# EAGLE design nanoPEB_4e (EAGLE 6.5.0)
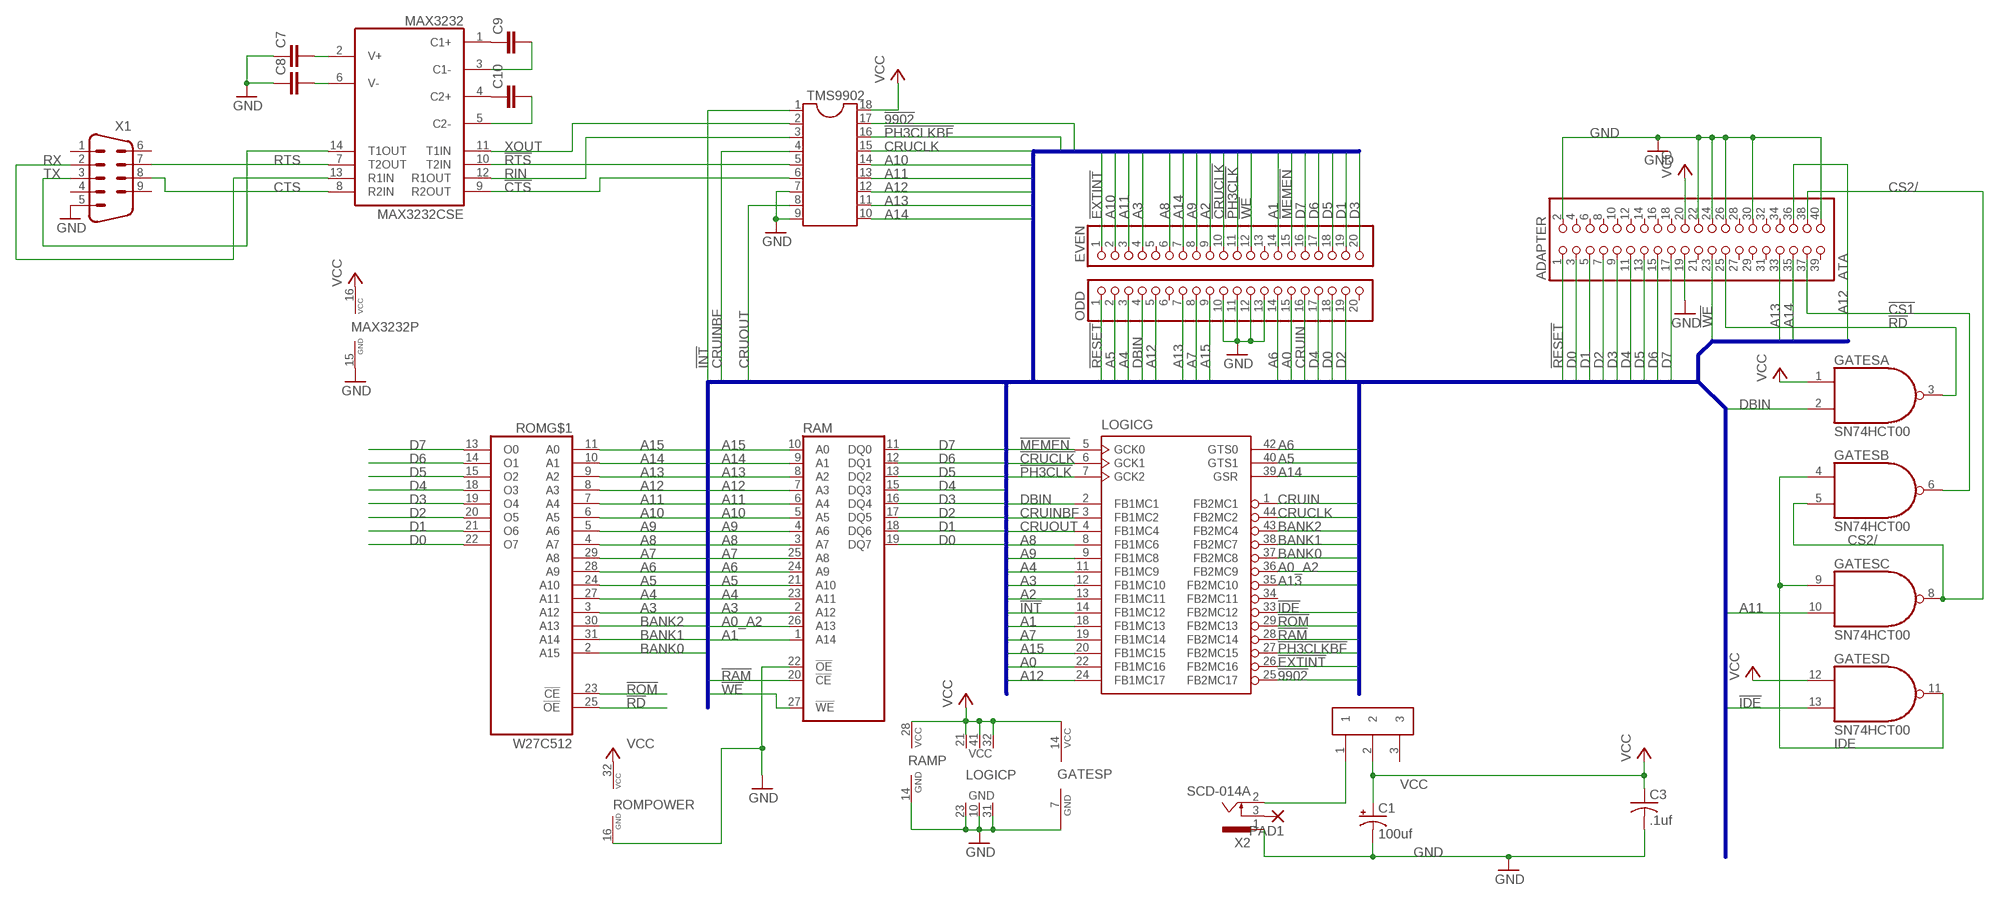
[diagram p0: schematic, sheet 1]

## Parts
ADAPTER  ATA  PINHD-2X20  [2X20]
C1  100uf  CPOL-USE2.5-6  [E2,5-6]
C3  .1uf  C-USC0805  [C0805]
C7  C-EUC0805  [C0805]
C8  C-EUC0805  [C0805]
C9  C-EUC0805  [C0805]
C10  C-EUC0805  [C0805]
EVEN  PINHD-1X20  [1X20]
GATES  SN74HCT00  74LS00D  [SO14]
LOGIC  XC9536-44PC44  [PC44]
MAX3232  MAX3232CSE  [SO16]
ODD  PINHD-1X20  [1X20]
PAD1  1,6/0,8  [1,6/0,8]
POWER  OS1020  [OS1020]
RAM  LH52256CHN  [SOP28]
ROM  W27C512  [PLCC32R-WINBOND]
TMS9902  DIL18S  [SOCKED-18]
X1  M09H  [M09H]
X2  SCD-014A  [SCD-014-A]

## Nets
!9902: LOGIC.25(G:FB2MC17) TMS9902.17
!CRUCLK: EVEN.10 LOGIC.6(G:GCK1)
!CS1: ADAPTER.37 GATES.6(B:O)
!CTS: MAX3232.9(R2OUT) TMS9902.6
!EXTINT: EVEN.1 LOGIC.26(G:FB2MC16)
!IDE: GATES.13(D:I1) LOGIC.33(G:FB2MC12)
!INT: LOGIC.14(G:FB1MC12) TMS9902.1
!MEMEN: EVEN.15 LOGIC.5(G:GCK0)
!PH3CLK: EVEN.11 LOGIC.7(G:GCK2)
!PH3CLKBF: LOGIC.27(G:FB2MC15) TMS9902.16
!RAM: LOGIC.28(G:FB2MC14) RAM.20(!CE)
!RD: ADAPTER.25 GATES.3(A:O) ROM.25(!OE)
!RESET: ADAPTER.1 ODD.1
!ROM: LOGIC.29(G:FB2MC13) ROM.23(!CE)
!RTS: MAX3232.10(T2IN) TMS9902.5
!WE: ADAPTER.23 EVEN.12 RAM.27(!WE)
A0: LOGIC.22(G:FB1MC16) ODD.15
A0_A2: LOGIC.36(G:FB2MC9) RAM.26(A13)
A1: EVEN.14 LOGIC.18(G:FB1MC13) RAM.1(A14)
A2: EVEN.9 LOGIC.13(G:FB1MC11)
A3: EVEN.4 LOGIC.12(G:FB1MC10) RAM.2(A12) ROM.3(A12)
A4: LOGIC.11(G:FB1MC9) ODD.3 RAM.23(A11) ROM.27(A11)
A5: LOGIC.40(G:GTS1) ODD.2 RAM.21(A10) ROM.24(A10)
A6: LOGIC.42(G:GTS0) ODD.14 RAM.24(A9) ROM.28(A9)
A7: LOGIC.19(G:FB1MC14) ODD.8 RAM.25(A8) ROM.29(A8)
A8: EVEN.6 LOGIC.8(G:FB1MC6) RAM.3(A7) ROM.4(A7)
A9: EVEN.8 LOGIC.9(G:FB1MC8) RAM.4(A6) ROM.5(A6)
A10: EVEN.2 RAM.5(A5) ROM.6(A5) TMS9902.14
A11: EVEN.3 GATES.10(C:I1) RAM.6(A4) ROM.7(A4) TMS9902.13
A12: ADAPTER.36 LOGIC.24(G:FB1MC17) ODD.5 RAM.7(A3) ROM.8(A3) TMS9902.12
A13: ADAPTER.33 LOGIC.35(G:FB2MC10) ODD.7 RAM.8(A2) ROM.9(A2) TMS9902.11
A14: ADAPTER.35 EVEN.7 LOGIC.39(G:GSR) RAM.9(A1) ROM.10(A1) TMS9902.10
A15: LOGIC.20(G:FB1MC15) ODD.9 RAM.10(A0) ROM.11(A0)
BANK0: LOGIC.37(G:FB2MC8) ROM.2(A15)
BANK1: LOGIC.38(G:FB2MC7) ROM.31(A14)
BANK2: LOGIC.43(G:FB2MC4) ROM.30(A13)
CRUCLK: LOGIC.44(G:FB2MC2) TMS9902.15
CRUIN: LOGIC.1(G:FB2MC1) ODD.16
CRUINBF: LOGIC.3(G:FB1MC2) TMS9902.4
CRUOUT: LOGIC.4(G:FB1MC4) TMS9902.8
CS2/: ADAPTER.38 GATES.5(B:I1) GATES.8(C:O)
CTS: MAX3232.8(R2IN) X1.8
D0: ADAPTER.3 ODD.18 RAM.19(DQ7) ROM.22(O7)
D1: ADAPTER.5 EVEN.19 RAM.18(DQ6) ROM.21(O6)
D2: ADAPTER.7 ODD.19 RAM.17(DQ5) ROM.20(O5)
D3: ADAPTER.9 EVEN.20 RAM.16(DQ4) ROM.19(O4)
D4: ADAPTER.11 ODD.17 RAM.15(DQ3) ROM.18(O3)
D5: ADAPTER.13 EVEN.18 RAM.13(DQ2) ROM.15(O2)
D6: ADAPTER.15 EVEN.17 RAM.12(DQ1) ROM.14(O1)
D7: ADAPTER.17 EVEN.16 RAM.11(DQ0) ROM.13(O0)
DBIN: GATES.2(A:I1) LOGIC.2(G:FB1MC1) ODD.4
GND [gnd]: ADAPTER.2 ADAPTER.19 ADAPTER.22 ADAPTER.24 ADAPTER.26 ADAPTER.30 ADAPTER.40 C1.- C3.2 C7.1 C8.1 GATES.7(P:GND) LOGIC.10(P:GND) LOGIC.23(P:GND) LOGIC.31(P:GND) MAX3232.15(GND) ODD.10 ODD.11 ODD.12 ODD.13 RAM.14(GND) RAM.22(!OE) ROM.16(POWER:GND) TMS9902.7 TMS9902.9 X1.5 X2.1
IDE: GATES.4(B:I0) GATES.9(C:I0) GATES.11(D:O)
N$1: C9.1 MAX3232.1(C1+)
N$2: C9.2 MAX3232.3(C1-)
N$3: C10.1 MAX3232.4(C2+)
N$5: PAD1.1(P) X2.3
N$6: POWER.1 X2.2
N$7: C8.2 MAX3232.6(V-)
N$8: C7.2 MAX3232.2(V+)
N$9: C10.2 MAX3232.5(C2-)
RIN: MAX3232.12(R1OUT) TMS9902.3
RTS: MAX3232.7(T2OUT) X1.7
RX: MAX3232.13(R1IN) X1.2
TX: MAX3232.14(T1OUT) X1.3
VCC [VCC]: ADAPTER.20 C1.+ C3.1 GATES.1(A:I0) GATES.12(D:I0) GATES.14(P:VCC) LOGIC.21(P:VCC) LOGIC.32(P:VCC) LOGIC.41(P:VCC) MAX3232.16(VCC) POWER.2 RAM.28(VCC) ROM.32(POWER:VCC) TMS9902.18
XOUT: MAX3232.11(T1IN) TMS9902.2
Unconnected: ADAPTER.4 ADAPTER.6 ADAPTER.8 ADAPTER.10 ADAPTER.12 ADAPTER.14 ADAPTER.16 ADAPTER.18 ADAPTER.21 ADAPTER.27 ADAPTER.28 ADAPTER.29 ADAPTER.31 ADAPTER.32 ADAPTER.34 ADAPTER.39 EVEN.5 EVEN.13 LOGIC.15(J:TDI) LOGIC.16(J:TMS) LOGIC.17(J:TCK) LOGIC.30(J:TDO) LOGIC.34(G:FB2MC11) ODD.6 ODD.20 POWER.3 ROM.1(NC1:NC) ROM.12(NC2:NC) ROM.17(NC3:NC) ROM.26(NC4:NC) X1.1 X1.4 X1.6 X1.9

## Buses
A[0..15],D[0..7],!MEMEN,!CRUCLK,CRUIN,!WE,DBIN,!IDE,!RAM,!ROM,!WE,A0_A2,BANK[0..2],!RESET,!9902,!EXTINT,!PH3CLK,!PH3CLKBF,CRUOUT,CRUCLK,CRUINBF,!INT

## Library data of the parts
ADAPTER = pinhead:PINHD-2X20: PIN HEADER
C1 = rcl:CPOL-US: POLARIZED CAPACITOR, American symbol
C3 = rcl:C-US: CAPACITOR, American symbol
C7-C10 = rcl:C-EU: CAPACITOR, European symbol
EVEN ODD = pinhead:PINHD-1X20: PIN HEADER
GATES = 74xx-us:74*00: Quad 2-input NAND gate
LOGIC = xilinx:XC9536-44
MAX3232 = maxim:MAX3232*: True RS-232 Transceivers 3.0V to 5.5V, Low-Power up to 1Mbps, Using Four 0.1µF External Capacitors Source: http://pdfserv.maxim-ic.com/en/ds/MAX3222-MAX3241.pdf; MPN: MAX3232CSE; OC_FARNELL: 9725490; OC_NEWARK: 90C2890
PAD1 = wirepad:1,6/0,8: THROUGH-HOLE PAD
POWER = OS1020:OS1020
RAM = memory-sram:LH52256CHN: MEMORY
ROM = am29-memory:W27C512
TMS9902 = ic-package:DIL18: Dual In Line
X1 = con-subd:M09: SUB-D
X2 = power_jack:SCD-014A: Power Jack 2.1mm

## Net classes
1 gnd: width 0.406 mm
2 VCC: width 0.406 mm

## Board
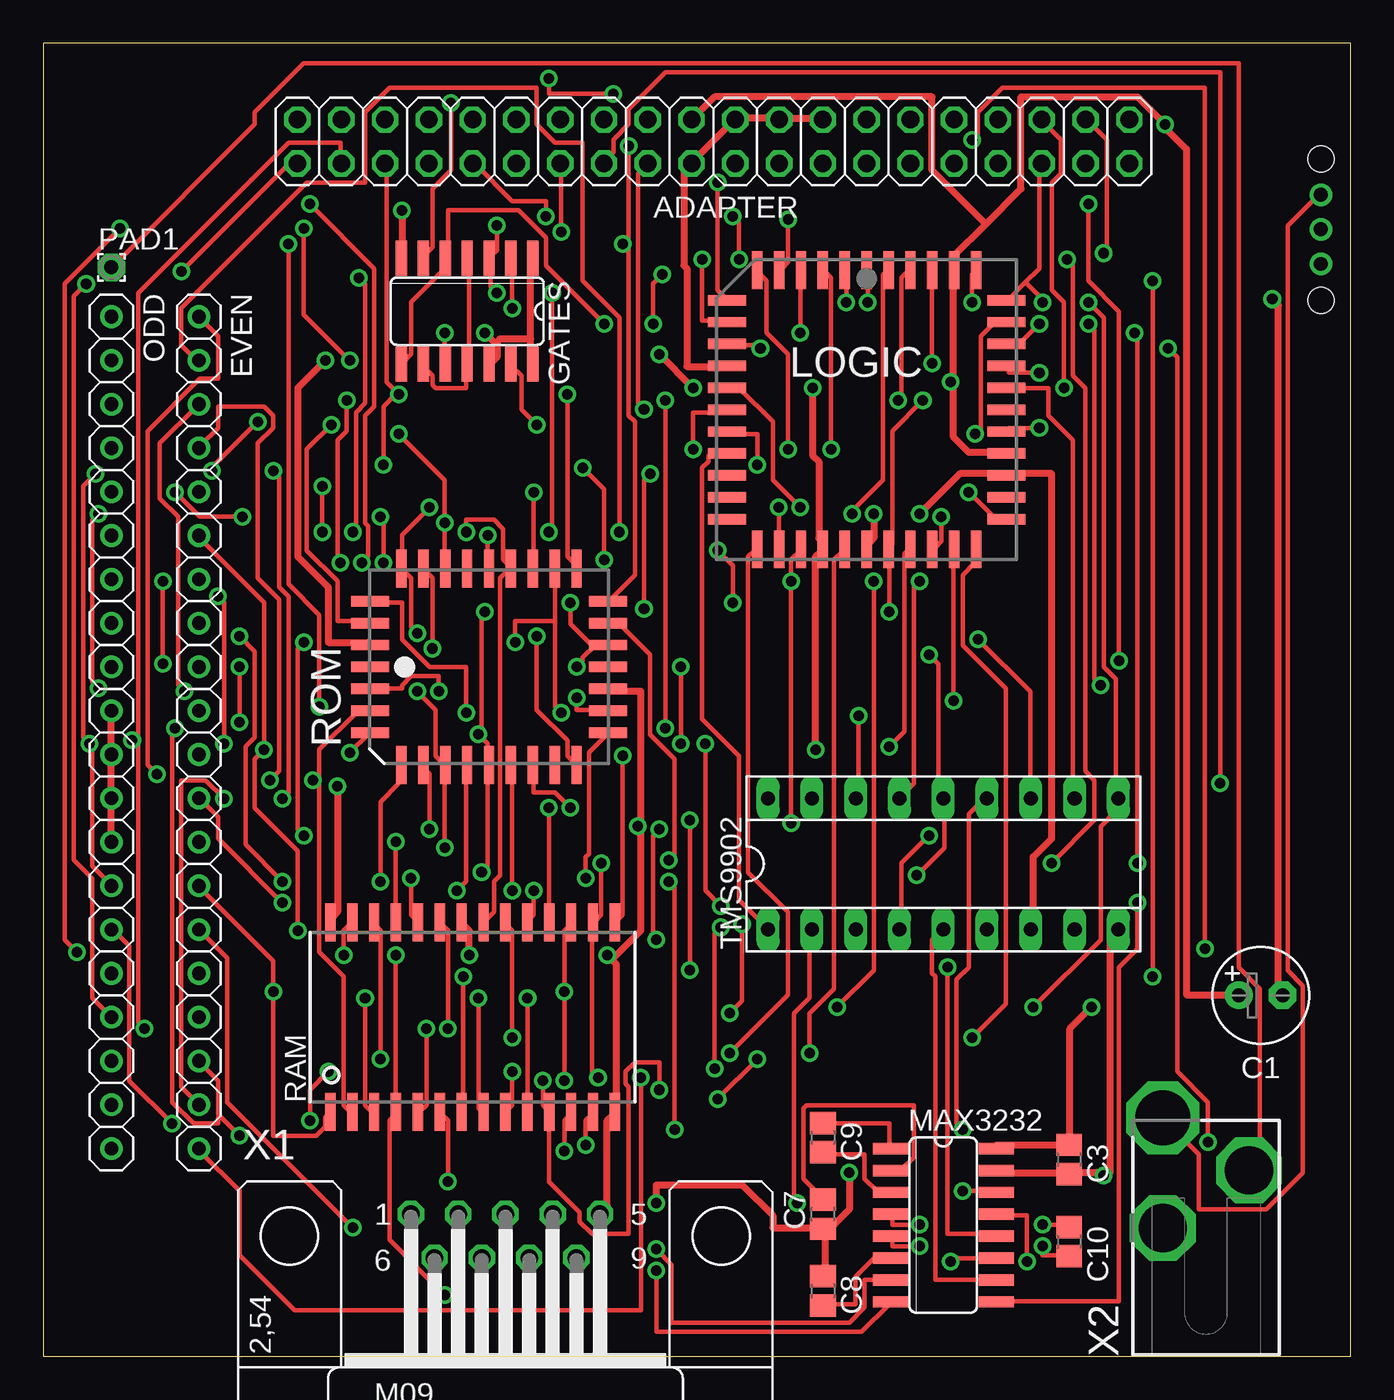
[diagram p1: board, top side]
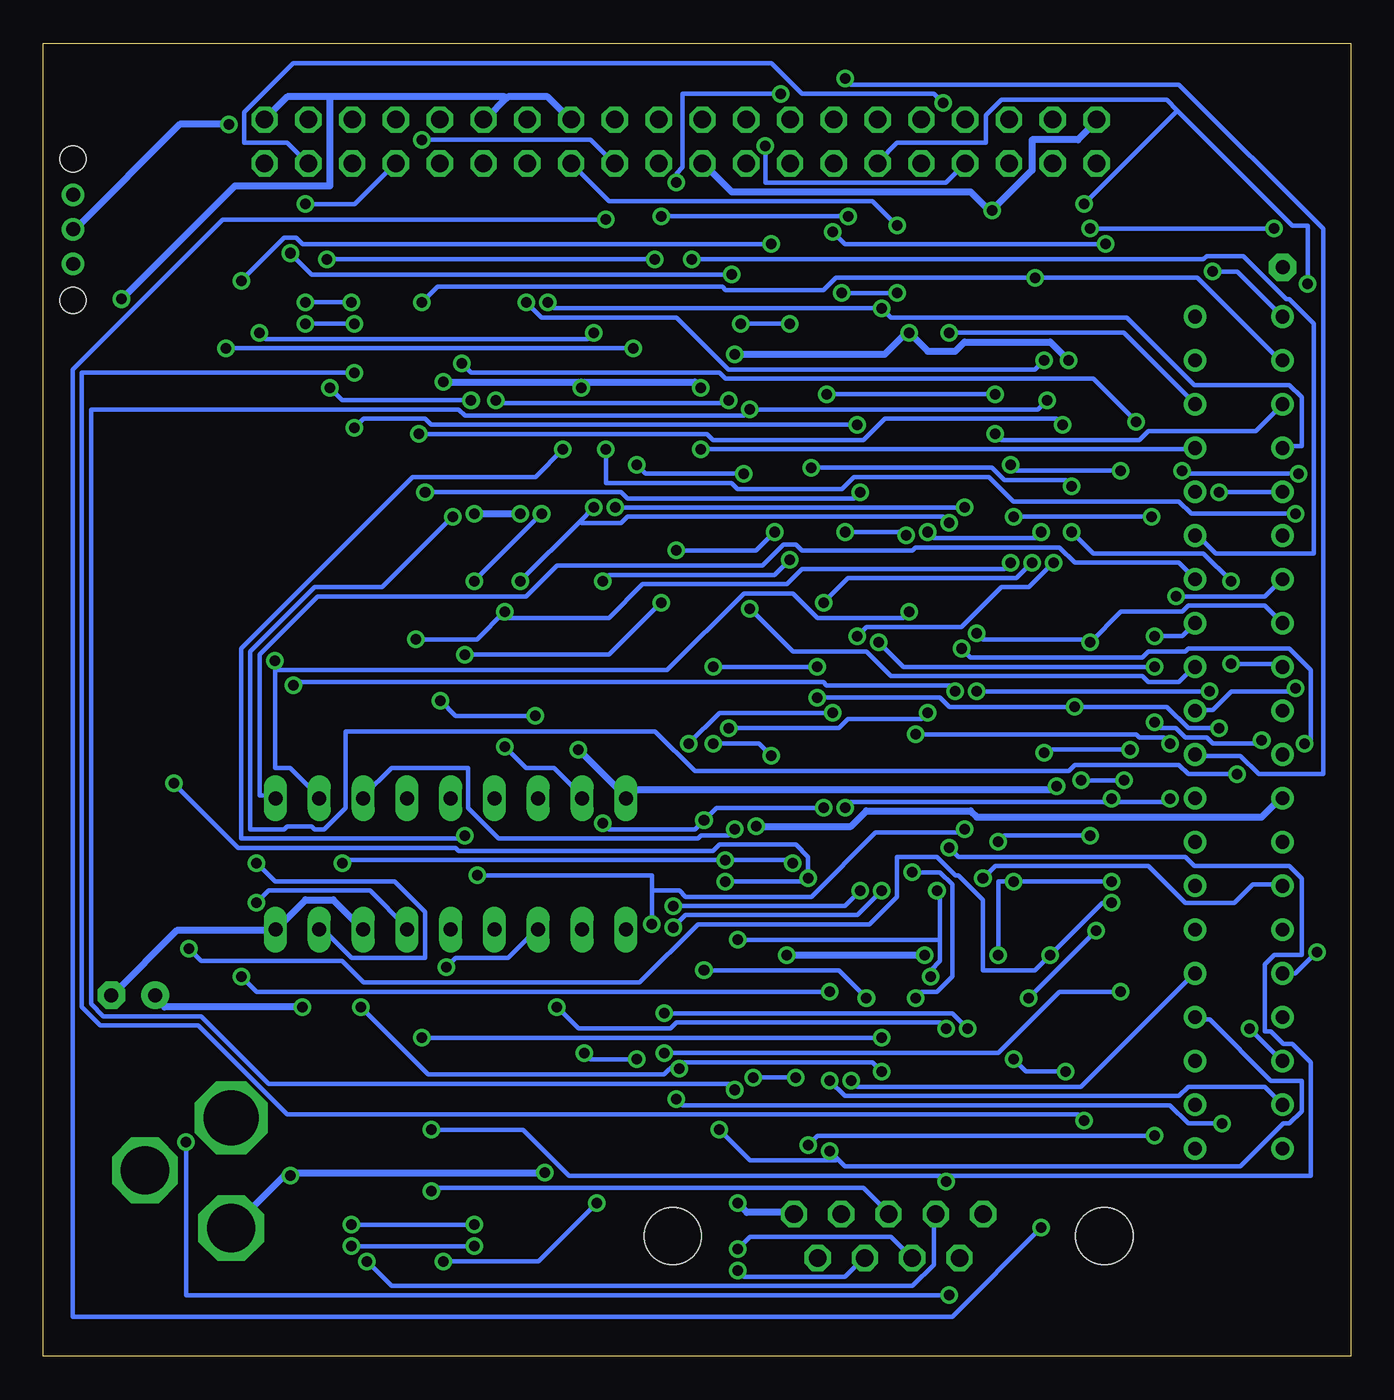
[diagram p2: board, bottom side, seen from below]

Size 75.87 x 76.19 mm. Coordinates in mm from the lower left corner, seen from the top.
Outline: 0,0 75.87,0 75.87,76.19 0,76.19 0,0
Copper layers (1*16): Top 0.035mm / dielectric 1.5mm / Bottom 0.035mm
Design rules "default": minimum track width 10mil, minimum drill 24mil, track to track 8mil, track to pad 8mil, pad to pad 8mil, via to via 8mil, smd to smd 8mil, copper to edge 40mil, drill to drill 8mil, minimum pad ring 10mil, minimum via ring 8mil, stop-mask expansion 4mil, vias tented up to drill 0mil, thermal gap 10mil

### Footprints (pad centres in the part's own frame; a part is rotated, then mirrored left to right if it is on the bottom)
2X20 = drill 1.016 octagon: 1 -24.13,-1.27; 2 -24.13,1.27; 3 -21.59,-1.27; 4 -21.59,1.27; 5 -19.05,-1.27; 6 -19.05,1.27; 7 -16.51,-1.27; 8 -16.51,1.27; 9 -13.97,-1.27; 10 -13.97,1.27; 11 -11.43,-1.27; 12 -11.43,1.27; 13 -8.89,-1.27; 14 -8.89,1.27; 15 -6.35,-1.27; 16 -6.35,1.27; 17 -3.81,-1.27; 18 -3.81,1.27; 19 -1.27,-1.27; 20 -1.27,1.27; 21 1.27,-1.27; 22 1.27,1.27; 23 3.81,-1.27; 24 3.81,1.27; 25 6.35,-1.27; 26 6.35,1.27; 27 8.89,-1.27; 28 8.89,1.27; 29 11.43,-1.27; 30 11.43,1.27; 31 13.97,-1.27; 32 13.97,1.27; 33 16.51,-1.27; 34 16.51,1.27; 35 19.05,-1.27; 36 19.05,1.27; 37 21.59,-1.27; 38 21.59,1.27; 39 24.13,-1.27; 40 24.13,1.27
E2,5-6 = drill 0.813 pad 1.6: + -1.27,0 | drill 0.813 pad 1.6 octagon: - 1.27,0
C0805 = smd 1.3 x 1.5: 1 -0.85,0; 2 0.85,0
1X20 = drill 0.8: 1 -24.13,0; 2 -21.59,0; 3 -19.05,0; 4 -16.51,0; 5 -13.97,0; 6 -11.43,0; 7 -8.89,0; 8 -6.35,0; 9 -3.81,0; 10 -1.27,0; 11 1.27,0; 12 3.81,0; 13 6.35,0; 14 8.89,0; 15 11.43,0; 16 13.97,0; 17 16.51,0; 18 19.05,0; 19 21.59,0; 20 24.13,0
SO14 = smd 0.66 x 2.032: 1 -3.81,-3.073; 2 -2.54,-3.073; 3 -1.27,-3.073; 4 0,-3.073; 5 1.27,-3.073; 6 2.54,-3.073; 7 3.81,-3.073; 8 3.81,3.073; 9 2.54,3.073; 10 1.27,3.073; 11 0,3.073; 12 -1.27,3.073; 13 -2.54,3.073; 14 -3.81,3.073
PC44 = smd 0.6 x 2.2: 1 0,8.1; 2 -1.27,8.1; 3 -2.54,8.1; 4 -3.81,8.1; 5 -5.08,8.1; 6 -6.35,8.1; 18 -6.35,-8.1; 19 -5.08,-8.1; 20 -3.81,-8.1; 21 -2.54,-8.1; 22 -1.27,-8.1; 23 0,-8.1; 24 1.27,-8.1; 25 2.54,-8.1; 26 3.81,-8.1; 27 5.08,-8.1; 28 6.35,-8.1; 40 6.35,8.1; 41 5.08,8.1; 42 3.81,8.1; 43 2.54,8.1; 44 1.27,8.1 | smd 2.2 x 0.6: 7 -8.1,6.35; 8 -8.1,5.08; 9 -8.1,3.81; 10 -8.1,2.54; 11 -8.1,1.27; 12 -8.1,0; 13 -8.1,-1.27; 14 -8.1,-2.54; 15 -8.1,-3.81; 16 -8.1,-5.08; 17 -8.1,-6.35; 29 8.1,-6.35; 30 8.1,-5.08; 31 8.1,-3.81; 32 8.1,-2.54; 33 8.1,-1.27; 34 8.1,0; 35 8.1,1.27; 36 8.1,2.54; 37 8.1,3.81; 38 8.1,5.08; 39 8.1,6.35
SO16 = smd 0.66 x 2.032: 1 -4.445,-3.073; 2 -3.175,-3.073; 3 -1.905,-3.073; 4 -0.635,-3.073; 5 0.635,-3.073; 6 1.905,-3.073; 7 3.175,-3.073; 8 4.445,-3.073; 9 4.445,3.073; 10 3.175,3.073; 11 1.905,3.073; 12 0.635,3.073; 13 -0.635,3.073; 14 -1.905,3.073; 15 -3.175,3.073; 16 -4.445,3.073
1,6/0,8 = drill 0.813 pad 1.6 octagon: 1 0,0
OS1020 = drill 0.8: 1 0,6.121; 2 0,4.115; 3 0,2.108 | hole 1.5: 0,0; 0,8.204
SOP28 = smd 0.6 x 2.2: 1 -8.255,-5.5; 2 -6.985,-5.5; 3 -5.715,-5.5; 4 -4.445,-5.5; 5 -3.175,-5.5; 6 -1.905,-5.5; 7 -0.635,-5.5; 8 0.635,-5.5; 9 1.905,-5.5; 10 3.175,-5.5; 11 4.445,-5.5; 12 5.715,-5.5; 13 6.985,-5.5; 14 8.255,-5.5; 15 8.255,5.5; 16 6.985,5.5; 17 5.715,5.5; 18 4.445,5.5; 19 3.175,5.5; 20 1.905,5.5; 21 0.635,5.5; 22 -0.635,5.5; 23 -1.905,5.5; 24 -3.175,5.5; 25 -4.445,5.5; 26 -5.715,5.5; 27 -6.985,5.5; 28 -8.255,5.5
PLCC32R-WINBOND = smd 0.6 x 2.2: 1 0,6.9; 2 -1.27,6.9; 3 -2.54,6.9; 4 -3.81,6.9; 14 -3.81,-6.9; 15 -2.54,-6.9; 16 -1.27,-6.9; 17 0,-6.9; 18 1.27,-6.9; 19 2.54,-6.9; 20 3.81,-6.9; 30 3.81,6.9; 31 2.54,6.9; 32 1.27,6.9 | smd 2.2 x 0.6: 5 -5.7,5.08; 6 -5.7,3.81; 7 -5.7,2.54; 8 -5.7,1.27; 9 -5.7,0; 10 -5.7,-1.27; 11 -5.7,-2.54; 12 -5.7,-3.81; 13 -5.7,-5.08; 21 5.7,-5.08; 22 5.7,-3.81; 23 5.7,-2.54; 24 5.7,-1.27; 25 5.7,0; 26 5.7,1.27; 27 5.7,2.54; 28 5.7,3.81; 29 5.7,5.08
SOCKED-18 = drill 0.813 long: 1 -10.16,-3.81; 2 -7.62,-3.81; 3 -5.08,-3.81; 4 -2.54,-3.81; 5 0,-3.81; 6 2.54,-3.81; 7 5.08,-3.81; 8 7.62,-3.81; 9 10.16,-3.81; 10 10.16,3.81; 11 7.62,3.81; 12 5.08,3.81; 13 2.54,3.81; 14 0,3.81; 15 -2.54,3.81; 16 -5.08,3.81; 17 -7.62,3.81; 18 -10.16,3.81
M09H = drill 1.016 octagon: 1 -5.486,1.27; 2 -2.743,1.27; 3 0,1.27; 4 2.743,1.27; 5 5.486,1.27; 6 -4.115,-1.27; 7 -1.372,-1.27; 8 1.372,-1.27; 9 4.115,-1.27 | hole 3.302: 12.522,0; -12.522,0
SCD-014-A = drill 2.8 pad 3.81 octagon: 1 -2.5,7.45; 3 2.5,10.8 | drill 3.2 pad 3.81 octagon: 2 -2.5,13.85

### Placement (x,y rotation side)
ADAPTER  38.89,70.48 0 top
C1  70.64,20.95 0 top
C3  59.52,11.42 270 top
C7  45.24,8.25 90 top
C8  45.24,3.81 270 top
C9  45.24,12.69 270 top
C10  59.52,6.66 270 top
EVEN  9.04,36.19 270 top
GATES  24.6,60.64 180 top
LOGIC  47.78,54.92 0 top
MAX3232  52.22,7.62 270 top
ODD  3.96,36.19 270 top
PAD1  3.96,63.18 0 top
POWER  74.13,61.27 0 top
RAM  24.92,19.68 0 top
ROM  25.87,40 90 top
TMS9902  52.22,28.57 0 top
X1  26.82,6.98 0 top
X2  67.46,-0.01 0 top

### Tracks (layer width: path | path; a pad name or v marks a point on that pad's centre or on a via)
!9902  (via drill 0.61)
  Top 0.254: v49.09,35.38 49.98,36.27 49.98,46.58 50.15,46.76 LOGIC.25
  Bottom 0.254: v49.09,35.38 47.84,34.13 46.24,34.13 44.64,32.53 TMS9902.17
!CRUCLK  (via drill 0.61)
  Top 0.254: v43.22,52.62 43.22,58.14 41.97,59.38 41.97,62.4 41.44,62.94 LOGIC.6 | v3.21,48.89 2.86,48.53 2.86,39.11 v3.21,38.75
  Bottom 0.254: v43.22,52.62 43.22,50.67 35.93,50.67 35.57,50.31 29.53,50.31 28.82,51.02 20.99,51.02 19.57,49.6 9.97,49.6 9.26,48.89 v3.21,48.89 | v3.21,38.75 3.39,38.58 6.95,38.58 8.01,37.51 8.9,37.51 EVEN.10
!CS1  (via drill 0.61)
  Top 0.254: v23.66,72.72 23.66,68.8 22.59,67.74 22.59,64.36 22.06,63.82 GATES.6
  Bottom 0.254: v23.66,72.72 24.19,73.25 31.84,73.25 33.62,75.03 61.35,75.03 64.2,72.18 64.2,70.4 61.71,70.4 60.64,69.34 ADAPTER.37
!CTS  (via drill 0.61)
  Top 0.254: v63.49,26.31 63.49,23.64 62.42,22.58 62.42,3.2 55.31,3.2 MAX3232.9
  Bottom 0.254: v63.49,26.31 62.78,27.02 56.91,27.02 54.77,24.89 TMS9902.6
!EXTINT  (via drill 0.61)
  Top 0.254: v52.11,48.71 52.11,47.29 51.75,46.93 LOGIC.26 | v6.59,33.78 6.06,34.31 6.06,53.69 9.08,56.71 10.15,56.71 10.15,59.2 9.08,60.27 EVEN.1
  Bottom 0.254: v52.11,48.71 56.2,44.62 60.11,44.62 63.84,40.89 63.84,30.58 61.89,30.58 61.71,30.75 60.29,30.75 60.11,30.58 59.58,30.58 58.33,31.82 58.33,36.27 40.37,36.27 38.06,33.95 16.37,33.95 16.02,34.31 9.97,34.31 9.44,33.78 v6.59,33.78
!IDE  (via drill 0.61)
  Top 0.254: v28.64,54.05 27.75,54.93 27.75,56.89 27.22,57.42 GATES.13 | v57.8,53.87 56.02,53.87 56.02,53.69 LOGIC.33
  Bottom 0.254: v28.64,54.05 53.35,54.05 53.71,54.4 57.26,54.4 v57.8,53.87
!INT
  Top 0.254: LOGIC.14 39.66,52.27 38.59,52.27 38.59,51.91 38.24,51.56 38.24,36.98 40.37,34.84 40.37,26.49 41.97,24.89 TMS9902.1
!MEMEN  (via drill 0.61)
  Top 0.254: v43.22,65.96 43.22,63.47 42.86,63.11 LOGIC.5 | v17.97,7.46 10.68,14.75 10.68,23.11 9.08,24.71 EVEN.15
  Bottom 0.254: v43.22,65.96 65.44,65.96 74.15,57.25 74.15,2.31 23.13,2.31 v17.97,7.46
!PH3CLK  (via drill 0.61)
  Top 0.254: v39.13,68.09 39.13,61.87 39.66,61.34 LOGIC.7 | v33.08,73.25 29.35,73.25 v29.35,74.14
  Bottom 0.254: v39.13,68.09 39.13,68.63 38.77,68.98 38.77,73.25 v33.08,73.25 | v29.35,74.14 28.99,73.78 9.97,73.78 1.61,65.43 1.61,33.78 5.35,33.78 6.41,34.84 8.9,34.84 EVEN.11
!PH3CLKBF  (via drill 0.61)
  Top 0.254: v52.82,38.04 52.82,46.76 LOGIC.27 | v47.31,37.15 47.31,32.53 TMS9902.16
  Bottom 0.254: v52.82,38.04 51.93,37.15 v47.31,37.15
!RAM  (via drill 0.61)
  Top 0.254: v27.22,18.49 27.22,24.71 26.86,25.07 RAM.20 | v53.89,18.49 55.84,20.44 55.84,38.75 53.35,41.24 53.35,45.33 54.06,46.04 54.06,46.76 LOGIC.28
  Bottom 0.254: v53.89,18.49 v27.22,18.49
!RD  (via drill 0.61)
  Top 0.254: v26.33,65.6 26.33,64.18 25.97,63.82 GATES.3 25.97,63.65 25.97,62.05 v26.33,61.69 | v25.79,47.64 25.79,45.87 ROM.25 | v29.35,47.82 29.53,48 v29.53,61.69
  Bottom 0.254: v26.33,65.6 27.75,67.03 43.04,67.03 45.17,69.16 ADAPTER.25 | v25.79,47.64 25.97,47.82 v29.35,47.82 | v26.33,61.69 v29.53,61.69
!RESET  (via drill 0.61)
  Top 0.254: v8.01,62.94 14.24,69.16 14.59,69.16 ADAPTER.1
  Bottom 0.254: v8.01,62.94 6.59,62.94 4.1,60.45 ODD.1
!ROM  (via drill 0.61)
  Top 0.254: v28.46,50.13 28.46,45.87 ROM.23 | v53.71,50.13 55.13,48.71 55.84,48.71 LOGIC.29
  Bottom 0.254: v28.46,50.13 28.82,49.78 41.97,49.78 42.33,50.13 v53.71,50.13
!RTS
  Top 0.254: MAX3232.10 51.75,4.44 51.75,22.04 51.58,22.22 51.58,24.18 52.11,24.71 TMS9902.5
!WE  (via drill 0.61)
  Top 0.254: v17.44,23.29 17.44,24.71 17.79,25.07 RAM.27 | v13.88,26.31 10.15,30.04 10.15,31.29 9.08,32.35 EVEN.12 | v53.89,70.58 54.24,70.94 54.24,72.18 55.66,73.6 67.4,73.6 v67.4,23.64
  Bottom 0.254: v13.88,26.31 14.42,26.31 v17.44,23.29 18.33,22.4 21.35,22.4 21.35,26.49 22.77,27.91 22.95,27.91 24.02,28.98 26.33,28.98 26.33,26.67 27.93,25.07 37.88,25.07 41.26,21.69 57.26,21.69 58.51,22.93 66.69,22.93 v67.4,23.64 | v53.89,70.58 44.11,70.58 42.86,69.34 ADAPTER.23
A0  (via drill 0.61)
  Top 0.254: v44.46,17.6 44.46,19.91 45.88,21.33 45.88,46.22 46.42,46.76 LOGIC.22 | v39.13,14.93 v41.44,17.24 | v7.48,13.51 4.99,16 4.99,23.82 4.1,24.71 ODD.15
  Bottom 0.254: v44.46,17.6 44.11,17.24 v41.44,17.24 | v39.13,14.93 38.77,14.57 10.5,14.57 9.44,13.51 v7.48,13.51
A0_A2  (via drill 0.61)
  Top 0.254: v19.57,17.24 19.57,24.71 19.21,25.07 RAM.26 | v16.55,16.53 15.48,15.46 v15.48,13.69 | v57.8,57.07 56.02,57.07 56.02,57.42 LOGIC.36
  Bottom 0.254: v19.57,17.24 18.86,16.53 v16.55,16.53 | v15.48,13.69 15.84,14.04 61.71,14.04 66.87,19.2 72.55,19.2 73.62,20.26 73.62,57.07 v57.8,57.07
A1  (via drill 0.61)
  Top 0.254: RAM.1 16.55,14.04 16.37,13.86 16.37,13.33 15.84,12.8 13.35,12.8 v13.35,21.15 13.35,22.93 9.08,27.2 EVEN.14 | v39.84,17.6 43.22,20.98 43.22,25.78 40.91,28.09 40.91,46.4 41.26,46.76 LOGIC.18
  Bottom 0.254: v39.84,17.6 20.46,17.6 16.9,21.15 v13.35,21.15
A2  (via drill 0.61)
  Top 0.254: v41.44,51.73 41.44,53.51 39.84,53.51 LOGIC.13 | v35.22,51.2 34.86,50.85 v34.86,43.38
  Bottom 0.254: v41.44,51.73 40.91,51.2 v35.22,51.2 | v34.86,43.38 32.37,40.89 28.11,40.89 26.68,39.47 12.1,39.47 11.75,39.11 9.97,39.11 9.08,40 EVEN.9
A3  (via drill 0.61)
  Top 0.254: 16.02,33.42 16.02,35.2 18.15,37.33 18.86,37.33 ROM.3 | 16.02,33.42 16.02,23.46 17.44,22.04 17.44,14.57 17.79,14.22 RAM.2 | v37.71,52.62 37.71,54.76 39.66,54.76 LOGIC.12 | v15.66,33.42 16.02,33.42 | v13.17,33.42 13.7,33.95 13.7,43.91 12.46,45.16 12.46,52.98 13.35,53.87 13.35,54.58 12.81,55.11 10.15,55.11 10.15,53.87 9.08,52.8 EVEN.4
  Bottom 0.254: v37.71,52.62 9.08,52.62 EVEN.4 | v13.17,33.42 v15.66,33.42
A4  (via drill 0.61)
  Top 0.254: v23.48,19.02 23.48,24.71 23.13,25.07 RAM.23 | v46.06,20.26 48.2,22.4 v48.2,44.98 | v43.93,49.25 42.33,50.85 42.33,54.22 40.37,56.18 39.84,56.18 LOGIC.11 | ROM.27 23.3,45.87 v23.3,48.36 23.3,50.85 v20.64,53.51
  Bottom 0.254: v23.48,19.02 23.84,19.38 39.13,19.38 39.48,19.02 44.82,19.02 v46.06,20.26 | v43.93,49.25 44.73,48.45 | 44.73,48.45 v48.2,44.98 | v23.3,48.36 23.66,48.71 41.97,48.71 42.33,48.36 44.64,48.36 44.73,48.45 | v20.64,53.51 20.28,53.16 12.28,53.16 11.75,53.69 5.53,53.69 4.1,55.11 ODD.3
A5  (via drill 0.61)
  Top 0.254: RAM.21 25.62,25.24 26.15,25.78 26.15,27.55 26.51,27.91 26.51,45.16 27.04,45.69 ROM.24 27.04,45.87 26.68,46.22 26.68,48 26.15,48.53 24.55,48.53 v24.55,47.82 | v53.89,61.16 53.89,62.76 54.06,62.94 LOGIC.40 | v17.97,47.82 18.15,48 18.15,54.76 18.68,55.29 18.68,62.22 v18.33,62.58
  Bottom 0.254: v53.89,61.16 53,62.05 36.46,62.05 36.28,61.87 30.59,61.87 29.88,62.58 v18.33,62.58 8.9,62.58 4.1,57.78 ODD.2 | v24.55,47.82 24.19,47.47 18.33,47.47 v17.97,47.82
A6  (via drill 0.61)
  Top 0.254: v21.35,27.73 21.35,25.6 21.7,25.24 RAM.24 | v22.59,41.07 22.59,45.16 22.06,45.69 ROM.28 | ODD.14 3.92,27.38 2.86,28.44 2.86,35.38 v2.68,35.55 2.32,35.91 2.32,50.49 v3.04,51.2 | v51.58,57.6 51.58,62.94 LOGIC.42 | v12.46,54.22 9.79,51.56 v9.79,51.38
  Bottom 0.254: v21.35,27.73 20.64,28.44 11.75,28.44 9.61,26.31 6.77,26.31 5.7,27.38 4.1,27.38 ODD.14 | v22.59,41.07 22.06,40.53 12.1,40.53 11.75,40.89 9.61,40.89 9.44,41.07 3.57,41.07 2.32,39.82 2.32,35.55 v2.68,35.55 | v51.58,57.6 51.04,57.07 36.64,57.07 36.28,56.71 14.95,56.71 v12.46,54.22 | v9.79,51.38 9.61,51.2 v3.04,51.2
A7  (via drill 0.61)
  Top 0.254: v20.46,29.87 20.46,25.24 RAM.25 | v15.13,30.22 14.77,30.58 14.77,41.07 v15.13,41.42 | v21.7,41.96 21.35,42.31 21.35,45.16 20.82,45.69 ROM.29 20.82,45.87 20.82,47.64 v22.42,49.25 | v42.69,49.25 42.69,46.93 LOGIC.19
  Bottom 0.254: v20.46,29.87 20.1,30.22 v15.13,30.22 | ODD.8 4.1,42.67 4.99,43.56 9.44,43.56 9.79,43.2 13.35,43.2 v15.13,41.42 15.13,41.6 21.35,41.6 v21.7,41.96 | v22.42,49.25 v42.69,49.25
A8  (via drill 0.61)
  Top 0.254: v17.79,35.02 18.86,36.09 ROM.4 | EVEN.6 9.08,47.47 12.81,43.73 v12.81,35.2 12.28,34.67 12.28,31.82 14.77,29.33 v14.77,24.71 | v18.68,20.8 18.68,14.57 19.04,14.22 RAM.3 | v38.24,63.65 38.24,60.09 39.66,60.09 LOGIC.8
  Bottom 0.254: v17.79,35.02 17.62,35.2 v12.81,35.2 | v14.77,24.71 v18.68,20.8 | v38.24,63.65 8.55,63.65 8.37,63.82 6.24,63.82 3.75,61.34 3.57,61.34 2.15,59.91 2.15,46.58 7.84,46.58 8.73,47.47 8.9,47.47 EVEN.6
A9  (via drill 0.61)
  Top 0.254: v20.46,23.29 20.46,14.22 RAM.4 20.46,14.04 20.1,13.69 20.1,6.75 v23.3,3.55 | v19.57,27.55 19.57,32.18 20.64,33.24 20.64,34.13 ROM.5 | v41.62,58.49 41.62,58.67 39.84,58.67 LOGIC.9 | v65.27,58.49 65.8,57.96 65.8,16.53 67.58,14.75 v67.58,12.44 | v11.39,41.78 12.28,40.89 12.28,35.91 11.75,35.38 11.75,29.69 v13.88,27.55
  Bottom 0.254: v20.46,23.29 20.46,27.55 v19.57,27.55 v13.88,27.55 | v65.27,58.49 v41.62,58.49 | v67.58,12.44 67.58,3.55 v23.3,3.55 | v11.39,41.78 9.79,41.78 9.08,42.49 EVEN.8
A10  (via drill 0.61)
  Top 0.254: v22.24,19.02 22.24,14.57 21.88,14.22 RAM.5 | v39.84,19.91 40.55,20.62 v40.55,25.07 | v50.69,27.91 52.29,29.51 52.29,32.35 TMS9902.14 52.11,32.53 51.93,32.71 51.93,40.18 v51.4,40.71 | v22.42,30.58 22.42,33.78 22.06,34.13 ROM.6 | v33.44,47.82 33.44,60.27 31.31,62.4 31.31,70.4 29.71,70.4 28.64,71.47 28.64,73.6 20.1,73.6 18.68,72.18 18.68,68.09 15.3,68.09 8.01,60.8 8.01,58.67 8.9,57.78 EVEN.2 | v39.13,46.76 40.02,45.87 v40.02,43.73
  Bottom 0.254: v22.24,19.02 23.13,19.91 v39.84,19.91 | 40.55,27.02 40.55,27.91 v50.69,27.91 | 40.55,27.02 v40.55,25.07 | v22.42,30.58 22.59,30.4 27.57,30.4 31.31,26.67 38.59,26.67 38.95,27.02 40.55,27.02 | v33.44,47.82 34.51,46.76 v39.13,46.76 | v40.02,43.73 43.04,40.71 v51.4,40.71
A11  (via drill 0.61)
  Top 0.254: v23.3,59.38 23.3,57.6 GATES.10 | v21.7,38.58 22.77,37.51 22.77,34.84 23.3,34.31 ROM.7 23.3,34.13 v23.3,29.51 | v8.19,38.58 7.84,38.93 7.84,48.71 6.77,49.78 6.77,52.98 8.9,55.11 EVEN.3 | v23.48,10.13 23.48,13.69 23.13,14.04 RAM.6 | v53.35,13.15 53,13.51 53,21.86 53.71,22.58 53.71,31.47 54.6,32.35 TMS9902.13
  Bottom 0.254: v23.3,59.38 13.17,59.38 9.08,55.29 EVEN.3 | v8.19,38.58 v21.7,38.58 | v53.35,13.15 48.02,13.15 45.35,10.48 23.84,10.48 v23.48,10.13 23.66,10.48 2.32,10.48 2.32,17.06 3.39,18.13 3.92,18.13 4.64,18.84 4.99,18.84 4.99,22.75 4.46,23.29 2.86,23.29 2.86,27.73 3.57,28.44 9.08,28.44 9.61,28.98 22.77,28.98 v23.3,29.51
A12  (via drill 0.61)
  Top 0.254: v24.37,22.04 24.37,14.22 RAM.7 | v24.02,27.02 24.55,27.55 24.55,34.13 ROM.8 | v49.09,43.2 49.09,46.76 LOGIC.24 49.09,46.93 49.26,47.11 49.26,53.69 v51.04,55.47 | v54.24,41.6 57.26,38.58 57.26,32.53 TMS9902.12 | v7.66,50.13 9.08,48.71 v11.57,48.71 | v19.57,48.71 19.75,48.53 v19.75,46.04 | v59.22,56.18 59.22,61.16 58.51,61.87 58.51,68.09 59.04,68.63 59.04,70.58 57.98,71.65 ADAPTER.36 | v35.57,24.18 35.4,24.35 35.4,30.22 v35.75,30.58
  Bottom 0.254: v24.37,22.04 24.37,22.4 23.84,22.93 23.84,24.18 | 23.84,24.18 23.84,27.02 v24.02,27.02 | v54.24,41.6 50.69,41.6 v49.09,43.2 49.26,42.84 43.04,42.84 41.09,44.8 32.73,44.8 31.84,45.69 20.1,45.69 v19.75,46.04 | v7.66,50.13 4.1,50.13 ODD.5 | v19.57,48.71 v11.57,48.71 | v59.22,56.18 58.51,55.47 v51.04,55.47 | v35.57,24.18 23.84,24.18 | v35.75,30.58 36.11,30.22 37.71,30.22 37.88,30.04 49.44,30.04 51.22,31.82 51.22,34.13 55.66,34.13 57.26,32.53 TMS9902.12
A13  (via drill 0.61)
  Top 0.254: LOGIC.35 56.02,56.18 58.33,56.18 58.33,54.58 59.75,53.16 59.75,32.53 TMS9902.11 | v60.64,66.85 60.64,62.4 62.42,60.62 v62.42,40.36 | v25.26,20.8 25.26,14.4 25.44,14.22 RAM.8 | v25.44,28.09 25.79,28.44 25.79,34.13 ROM.9 25.79,34.31 25.79,35.55 v25.26,36.09 25.44,36.09 25.44,43.02 v25.62,43.2 | v10.15,44.09 10.5,43.73 v10.5,35.55
  Bottom 0.254: v60.64,66.85 57.8,66.85 55.49,69.16 ADAPTER.33 | 62.42,39.82 62.42,34.13 61.53,34.13 59.93,32.53 TMS9902.11 | 62.42,39.82 v62.42,40.36 | v25.26,20.8 24.91,21.15 24.02,21.15 23.13,22.04 23.13,27.38 23.84,28.09 v25.44,28.09 | v10.15,44.09 4.99,44.09 4.1,44.98 ODD.7 | v10.5,35.55 10.86,35.91 12.28,35.91 12.46,36.09 v25.26,36.09 | 62.42,39.82 39.66,39.82 35.22,44.27 32.37,44.27 30.95,42.84 25.97,42.84 v25.62,43.2
A14  (via drill 0.61)
  Top 0.254: 57,62.31 57.8,63.11 57.8,69.16 ADAPTER.35 | 57,62.31 56.02,61.34 LOGIC.39 | v27.22,16.53 27.22,14.57 26.86,14.22 RAM.9 | v57.44,20.26 61.35,24.18 61.35,30.75 62.24,31.64 62.24,32.35 TMS9902.10 62.24,32.53 62.24,39.29 61.53,40 61.53,60.27 v60.64,61.16 | v27.22,27.02 27.22,34.13 ROM.10 | v39.31,24.89 38.95,24.53 v38.95,16.71 | 57,62.31 57.98,61.34 v57.98,61.16
  Bottom 0.254: v27.22,16.53 27.75,17.06 39.13,17.06 39.22,16.98 | 39.22,16.98 39.84,16.35 53.53,16.35 v57.44,20.26 | v27.22,27.02 28.64,25.6 38.59,25.6 v39.31,24.89 | 39.22,16.98 v38.95,16.71 | EVEN.7 9.08,45.16 9.97,46.04 16.02,46.04 16.9,46.93 25.26,46.93 25.44,46.76 31.84,46.76 32.2,47.11 32.91,47.11 34.15,45.87 46.06,45.87 47.84,44.09 59.93,44.09 63.31,40.71 63.31,32.53 62.42,32.53 TMS9902.10 | v60.64,61.16 v57.98,61.16
A15  (via drill 0.61)
  Top 0.254: v28.11,20.8 28.11,14.22 RAM.10 | v37.53,31.11 v37.53,22.4 | v30.59,31.82 29.71,32.71 28.46,32.71 28.46,34.13 ROM.11 | v43.4,30.93 v43.4,44.98 43.4,46.22 43.93,46.76 LOGIC.20 | v6.95,44.98 v6.95,40.18 | v16.19,50.49 v16.19,47.82 | v31.31,51.56 32.55,50.31 v32.55,46.22
  Bottom 0.254: v28.11,20.8 29.71,22.4 v37.53,22.4 | v30.59,31.82 36.82,31.82 v37.53,31.11 38.06,30.58 43.04,30.58 v43.4,30.93 | v6.95,40.18 4.28,40.18 4.1,40 ODD.9 | v6.95,44.98 8.55,46.58 14.95,46.58 v16.19,47.82 | v16.19,50.49 16.55,50.85 20.1,50.85 20.82,51.56 v31.31,51.56 | v32.55,46.22 33.44,45.33 43.04,45.33 v43.4,44.98
BANK0  (via drill 0.61)
  Top 0.254: v22.95,38.58 22.95,39.47 21.35,39.47 20.82,38.93 20.82,38.75 19.04,38.75 ROM.2 | v61.35,38.93 61,39.29 61,59.56 v60.64,59.91 | v57.8,59.91 56.73,58.85 56.02,58.85 LOGIC.37
  Bottom 0.254: v22.95,38.58 23.3,38.93 30.42,38.93 30.59,39.11 61.18,39.11 v61.35,38.93 | v57.8,59.91 v60.64,59.91
BANK1  (via drill 0.61)
  Top 0.254: v16.73,54.05 15.3,52.62 15.3,46.76 17.08,44.98 17.08,42.67 18.86,42.67 ROM.31 | v54.06,53.51 54.42,53.87 54.42,59.2 55.13,59.91 55.84,59.91 LOGIC.38
  Bottom 0.254: v16.73,54.05 17.08,54.4 27.04,54.4 28.28,53.16 36.99,53.16 37.35,53.51 v54.06,53.51
BANK2  (via drill 0.61)
  Top 0.254: v24.55,37.33 24.55,40 22.42,40 20.82,41.6 20.82,43.73 19.04,43.73 ROM.30 | v36.11,55.47 v36.11,36.44 | v49.62,55.47 49.8,55.65 49.8,62.58 50.15,62.94 LOGIC.43
  Bottom 0.254: v24.55,37.33 24.91,36.98 29.17,36.98 29.71,36.44 v36.11,36.44 | v36.11,55.47 36.28,55.29 49.44,55.29 v49.62,55.47
CRUCLK  (via drill 0.61)
  Top 0.254: v46.95,48.89 46.95,49.07 48.73,50.85 48.73,62.76 48.91,62.94 LOGIC.44 | v50.86,44.98 50.51,44.62 50.51,33.24 49.8,32.53 TMS9902.15
  Bottom 0.254: v50.86,44.98 v46.95,48.89
CRUIN  (via drill 0.61)
  Top 0.254: v47.84,61.16 47.84,62.94 LOGIC.1 | v17.79,57.78 15.13,60.45 v15.13,65.43 | v4.46,65.43 1.26,62.22 1.26,24.18 v1.97,23.46
  Bottom 0.254: v47.84,61.16 46.95,60.27 39.13,60.27 36.11,57.25 18.33,57.25 v17.79,57.78 | v4.46,65.43 v15.13,65.43 | v1.97,23.46 3.21,22.22 ODD.16
CRUINBF  (via drill 0.61)
  Top 0.254: v45.71,52.62 45.71,62.58 45.35,62.94 LOGIC.3 | v51.4,30.22 49.8,28.62 49.8,24.89 TMS9902.4
  Bottom 0.254: v45.71,52.62 47.31,51.02 54.42,51.02 64.38,41.07 64.38,30.04 51.58,30.04 v51.4,30.22
CRUOUT  (via drill 0.61)
  Top 0.254: v43.93,59.38 43.93,62.94 LOGIC.4 | v63.31,59.38 63.49,59.2 v63.49,28.62
  Bottom 0.254: v43.93,59.38 44.29,59.02 62.95,59.02 v63.31,59.38 | v63.49,28.62 62.42,27.55 55.49,27.55 53.71,25.78 53.71,23.11 57.98,23.11 59.58,24.71 59.75,24.71 TMS9902.8
CS2/  (via drill 0.61)
  Top 0.254: GATES.8 20.82,57.6 21.35,58.14 21.35,61.16 23.3,63.11 23.3,63.65 GATES.5 23.48,63.82 23.48,66.49 27.57,66.49 29.17,64.89 29.17,63.29 v32.55,59.91 | v61.53,64 61.71,64.18 61.71,70.58 60.64,71.65 ADAPTER.38 | v35.93,62.76 35.4,62.22 v35.4,59.91
  Bottom 0.254: v61.53,64 60.29,62.76 v35.93,62.76 | v32.55,59.91 v35.4,59.91
CTS  (via drill 0.61)
  Top 0.254: v35.57,4.97 35.57,1.42 47.48,1.42 49.09,3.02 MAX3232.8
  Bottom 0.254: v35.57,4.97 35.22,4.62 29.35,4.62 28.28,5.69 X1.8
D0  (via drill 0.61)
  Top 0.254: v28.46,27.02 28.46,25.6 28.11,25.24 RAM.19 | v39.31,26.13 38.42,27.02 v38.42,35.55 | v30.06,37.33 29.71,37.69 29.71,42.67 | 29.71,42.67 29.71,45.69 ROM.22 | v5.88,19.02 5.53,19.38 5.53,35.73 | 5.53,35.73 5.53,61.69 14.24,70.4 17.26,70.4 17.26,69.34 ADAPTER.3 | 29.71,42.67 27.39,42.67 v27.39,41.42 | v11.39,36.8 v11.39,40 | 5.53,35.73 v5.17,35.73
  Bottom 0.254: v28.46,27.02 29.35,26.13 v39.31,26.13 | v38.42,35.55 36.64,37.33 v30.06,37.33 | v5.88,19.02 4.1,17.24 ODD.18 | v27.39,41.42 25.97,40 v11.39,40 | v11.39,36.8 11.04,36.44 10.15,36.44 9.61,35.91 8.37,35.91 8.01,35.55 5.35,35.55 v5.17,35.73
D1  (via drill 0.61)
  Top 0.254: v30.42,55.82 30.42,46.4 30.95,45.87 ROM.21 | ADAPTER.5 19.93,69.16 19.93,56.53 v20.64,55.82 20.46,55.82 19.75,55.11 v19.75,51.73 | v29.35,31.82 29.35,25.24 RAM.18 | v10.5,32.35 9.44,33.42 8.01,33.42 8.01,15.64 8.9,14.75 EVEN.19 | v13.35,51.38 13.7,51.02 13.7,44.62 14.24,44.09 14.24,32.71 v13.88,32.35
  Bottom 0.254: v20.64,55.82 v30.42,55.82 | v29.35,31.82 28.99,32.18 13.88,32.18 | 13.88,32.18 10.68,32.18 v10.5,32.35 | v19.75,51.73 19.39,51.38 v13.35,51.38 | 13.88,32.18 v13.88,32.35
D2  (via drill 0.61)
  Top 0.254: v33.97,70.23 33.97,64.54 | 33.97,64.54 33.97,54.58 34.33,54.22 34.33,45.33 32.91,43.91 ROM.20 | v30.24,16 v30.24,21.15 30.24,24.71 30.59,25.07 RAM.17 | v33.62,64.54 33.97,64.54 | v64.38,22.04 v64.38,62.4
  Bottom 0.254: v33.97,70.23 33.97,68.09 23.48,68.09 22.42,69.16 ADAPTER.7 | v30.24,16 29.35,15.11 9.97,15.11 9.44,15.64 4.99,15.64 4.1,14.75 ODD.19 | v33.62,64.54 60.82,64.54 61.18,64.89 61.89,64.89 v64.38,62.4 | v64.38,22.04 63.49,21.15 v30.24,21.15
D3  (via drill 0.61)
  Top 0.254: v32.37,28.62 32.37,25.6 32.02,25.24 RAM.16 31.84,25.07 31.84,16.53 v32.2,16.18 | v36.28,28.8 36.64,29.15 36.64,34.67 35.22,36.09 35.22,40.71 33.44,42.49 32.91,42.49 ROM.19 | v34.68,16.18 34.68,2.66 14.59,2.66 11.39,5.86 11.39,9.6 9.08,11.91 EVEN.20 | v29.17,66.14 29.17,67.03 27.22,67.03 25.08,69.16 ADAPTER.9 | v40.02,66.14 40.37,65.78 v40.37,63.65 | v59.4,63.65 59.75,63.29 59.75,56.89 60.47,56.18 60.47,33.95 61,33.42 61,31.11 v58.51,28.62
  Bottom 0.254: v32.37,28.62 32.55,28.8 v36.28,28.8 58.33,28.8 v58.51,28.62 | v32.2,16.18 v34.68,16.18 | v40.02,66.14 v29.17,66.14 | v59.4,63.65 v40.37,63.65
D4  (via drill 0.61)
  Top 0.254: v33.62,34.84 33.62,25.6 33.26,25.24 RAM.15 | v36.99,40 v36.99,35.55 | v30.95,40 31.31,40.36 31.31,40.53 32.02,41.24 32.73,41.24 ROM.18 31.84,41.24 30.59,42.49 v30.59,43.73 | v2.5,62.22 1.79,61.51 1.79,28.8 2.86,27.73 2.86,20.8 3.92,19.73 ODD.17 | v18.5,46.04 18.86,46.4 18.86,48.18 18.68,48.36 18.68,54.58 19.21,55.11 19.21,63.11 v15.48,66.85
  Bottom 0.254: v33.62,34.84 34.33,35.55 v36.99,35.55 | v30.95,40 v36.99,40 | v2.5,62.22 2.5,65.6 3.39,65.6 10.06,72.27 | 10.06,72.27 10.68,72.89 20.28,72.89 21.17,72 21.17,70.4 26.33,70.4 27.39,69.34 ADAPTER.11 | v30.59,43.73 29.17,45.16 19.39,45.16 v18.5,46.04 | 10.06,72.27 v15.48,66.85
D5  (via drill 0.61)
  Top 0.254: v31.48,12.26 31.48,13.69 31.84,14.04 RAM.13 | 10.24,13.95 10.15,14.04 10.15,16 9.08,17.06 EVEN.18 | 10.24,13.95 v11.39,12.8 | v30.95,38.22 30.95,37.51 32.73,37.51 ROM.15 | v7.66,36.44 7.48,36.27 7.48,14.75 8.73,13.51 10.15,13.51 10.15,13.86 10.24,13.95 | v30.06,65.25 30.06,69.16 ADAPTER.13 | v14.24,64.54 14.24,44.8 16.02,43.02 v16.02,37.69
  Bottom 0.254: v31.48,12.26 30.95,12.8 v11.39,12.8 | v30.95,38.22 23.84,38.22 23.3,37.69 v16.02,37.69 10.68,37.69 9.44,36.44 v7.66,36.44 | v30.06,65.25 29.35,64.54 v14.24,64.54
D6  (via drill 0.61)
  Top 0.254: v30.24,11.91 30.24,13.69 30.59,14.04 RAM.12 | v31.48,27.73 31.48,28.98 31.66,29.15 31.66,35.02 32.73,36.09 ROM.14 | v36.28,27.55 36.64,27.2 v36.64,13.15 | v68.29,33.24 68.29,74.49 36.11,74.49 33.97,72.36 33.97,71.47 33.08,70.58 33.08,69.87 32.55,69.34 ADAPTER.15
  Bottom 0.254: 29.79,11.46 29.35,11.02 6.41,11.02 3.92,13.51 3.57,13.51 2.86,14.22 2.86,16 4.64,16 8.19,19.55 8.9,19.55 EVEN.17 | 29.79,11.46 v30.24,11.91 | v36.28,27.55 31.66,27.55 v31.48,27.73 31.48,28.98 32.2,29.69 36.64,29.69 36.99,29.33 51.75,29.33 51.93,29.51 64.55,29.51 v68.29,33.24 | v36.64,13.15 34.86,11.37 29.88,11.37 29.79,11.46
D7  (via drill 0.61)
  Top 0.254: v28.99,16 28.99,14.57 29.35,14.22 RAM.11 29.35,14.04 29.35,10.13 31.13,8.35 31.13,7.82 31.84,7.11 33.97,7.11 33.97,15.64 33.8,15.82 33.8,16.53 34.33,17.06 35.75,17.06 v35.75,15.46 | v28.64,41.78 28.64,37.51 30.42,35.73 30.42,34.84 30.95,34.31 ROM.13 | v17.26,46.04 17.08,46.22 17.08,53.16 17.62,53.69 v17.62,55.47 | v34.86,54.93 34.51,55.29 34.51,68.63 35.04,69.16 ADAPTER.17
  Bottom 0.254: v28.99,16 28.64,15.64 15.66,15.64 9.08,22.22 EVEN.16 | v28.64,41.78 28.11,42.31 22.59,42.31 20.28,44.62 18.68,44.62 v17.26,46.04 | v17.62,55.47 18.15,54.93 v34.86,54.93 35.22,54.58 51.4,54.58 51.75,54.93 73.09,54.93 73.09,20.44 72.38,19.73 66.69,19.73 62.78,15.82 36.11,15.82 v35.75,15.46
DBIN  (via drill 0.61)
  Top 0.254: v27.22,60.8 27.22,63.65 GATES.2 | v46.6,61.16 46.6,62.94 LOGIC.2
  Bottom 0.254: ODD.4 3.92,52.8 2.86,52.8 2.86,55.65 3.57,56.36 9.08,56.36 12.99,60.27 26.68,60.27 v27.22,60.8 46.24,60.8 v46.6,61.16
GND  (via drill 0.61)
  Top 0.406: ODD.13 3.92,29.87 3.92,32.35 ODD.12 3.92,32.53 3.92,34.84 ODD.11 3.92,35.02 3.92,37.33 ODD.10 | C8.1 45.35,4.8 45.35,7.29 C7.1 | 33.26,14.22 RAM.14 | RAM.14 33.08,14.04 32.73,13.69 32.73,8.71 32.37,8.35 X1.5 | v24.73,23.29 24.73,24.71 24.37,25.07 RAM.22 | RAM.14 33.26,14.4 33.26,22.75 v32.73,23.29 33.08,23.11 34.68,24.71 34.68,30.75 | 34.68,30.75 34.68,38.58 32.91,38.58 ROM.16 | v35.57,8.88 35.57,9.95 40.55,9.95 42.33,8.17 42.33,7.46 45.17,7.46 C7.1 | v34.51,30.75 34.68,30.75 | v20.82,66.49 20.82,63.82 GATES.7 | 39.66,57.42 LOGIC.10 39.48,57.42 37.35,57.42 37.35,63.11 37.17,63.29 37.17,68.8 37.53,69.16 ADAPTER.19 37.71,69.34 40.02,71.65 ADAPTER.22 40.2,71.83 42.69,71.83 ADAPTER.24 42.86,71.83 45.17,71.83 ADAPTER.26 | 47.84,46.93 LOGIC.23 47.84,47.11 48.2,47.47 v48.2,48.89 | v50.86,48.89 53.18,51.2 55.84,51.2 LOGIC.31 | 56.02,51.2 LOGIC.31 | 55.31,10.84 MAX3232.15 55.31,10.66 59.4,10.66 C3.2 59.58,10.66 61.53,10.66 | 61.53,10.66 61.89,10.66 61.89,24.35 62.24,24.71 TMS9902.9 | LOGIC.31 56.2,51.2 58.51,51.2 58.51,30.04 57.44,28.98 57.44,24.89 TMS9902.7 | v61.53,10.48 61.53,10.66 | v71.31,61.34 71.67,60.98 71.67,21.15 71.84,20.98 C1.- | v46.77,10.66 46.77,8.53 45.53,7.29 C7.1
  Bottom 0.406: v32.73,23.29 v24.73,23.29 | v35.57,8.88 35.04,8.35 32.37,8.35 X1.5 | v34.51,30.75 28.99,30.75 28.11,31.64 22.06,31.64 21.7,31.29 5.17,31.29 4.1,32.35 ODD.12 | ADAPTER.2 14.77,71.65 15.84,70.58 18.5,70.58 18.5,68.8 v20.82,66.49 20.99,66.49 22.06,67.56 35.93,67.56 37.53,69.16 ADAPTER.19 | 49,72.98 48.91,73.07 46.6,73.07 45.35,71.83 ADAPTER.26 | 49,72.98 50.15,71.83 ADAPTER.30 | 59.22,73.07 49.09,73.07 49,72.98 | 59.22,73.07 61.71,73.07 62.95,71.83 ADAPTER.40 | v50.86,48.89 v48.2,48.89 | TMS9902.7 57.44,24.89 59.04,26.49 60.64,26.49 62.24,24.89 TMS9902.9 62.42,24.71 68.11,24.71 71.84,20.98 C1.- | X2.1 64.91,7.46 61.89,10.48 v61.53,10.48 61.53,10.66 v46.77,10.66 | 59.22,73.07 59.22,67.92 64.73,67.92 v71.31,61.34
IDE
  Top 0.254: GATES.9 22.06,57.42 22.59,56.89 22.59,56.36 22.77,56.18 24.55,56.18 24.55,57.42 GATES.11 24.73,57.6 24.73,63.65 GATES.4
N$1
  Top 0.254: C9.1 45.35,13.51 49.09,13.51 49.09,12.08 MAX3232.1
N$2
  Top 0.254: C9.2 45.35,11.73 47.66,11.73 47.66,10.31 48.37,9.6 49.09,9.6 MAX3232.3
N$3  (via drill 0.61)
  Top 0.254: v57.98,7.64 59.4,7.64 C10.1 | v50.86,7.64 49.26,7.64 49.26,8.17 MAX3232.4
  Bottom 0.254: v50.86,7.64 v57.98,7.64
N$5
  Top 0.254: PAD1.1 4.1,63.29 12.28,71.47 12.28,72.18 15.13,75.03 69.35,75.03 69.35,22.58 70.6,21.33 70.6,11.37 70.07,10.84 X2.3
N$6
  Top 0.254: POWER.1 73.98,67.38 72.2,65.6 72.2,22.4 73.09,21.51 73.09,10.66 70.95,8.53 67.04,8.53 67.04,11.73 65.09,13.69 X2.2
N$7
  Top 0.254: C8.2 45.35,3.02 47.13,3.02 47.13,4.62 48.2,5.69 49.09,5.69 MAX3232.6
N$8
  Top 0.254: C7.2 45.17,9.24 44.11,10.31 44.11,14.4 44.29,14.57 50.51,14.57 50.51,11.55 49.8,10.84 49.26,10.84 MAX3232.2
N$9  (via drill 0.61)
  Top 0.254: v57.98,6.4 57.98,5.86 59.4,5.86 C10.2 | v50.86,6.4 49.26,6.4 49.26,6.93 MAX3232.5
  Bottom 0.254: v50.86,6.4 v57.98,6.4
RIN  (via drill 0.61)
  Top 0.254: v52.46,22.58 52.46,7.11 55.13,7.11 MAX3232.12
  Bottom 0.254: v52.46,22.58 51.93,23.11 48.91,23.11 47.31,24.71 TMS9902.3
RTS  (via drill 0.61)
  Top 0.254: MAX3232.7 47.66,4.44 47.66,2.84 46.77,1.95 36.46,1.95 36.46,5.33 v35.57,6.22
  Bottom 0.254: v35.57,6.22 34.86,6.93 26.68,6.93 25.62,5.86 X1.7
RX  (via drill 0.61)
  Top 0.254: v57.09,5.51 57.09,8.17 55.31,8.17 MAX3232.13
  Bottom 0.254: v57.09,5.51 55.66,4.08 25.44,4.08 24.19,5.33 24.19,8.17 X1.2
TX  (via drill 0.61)
  Top 0.254: v53.35,9.6 55.13,9.6 MAX3232.14
  Bottom 0.254: v53.35,9.6 53.18,9.77 28.28,9.77 26.86,8.35 X1.3
VCC  (via drill 0.61)
  Top 0.406: 45.35,46.93 LOGIC.21 | 16.73,25.24 RAM.28 16.73,25.42 17.08,25.78 v17.08,33.07 | v44.82,35.2 44.82,46.4 45.17,46.76 LOGIC.21 | 19.04,41.24 ROM.32 18.86,41.42 16.55,41.42 16.55,44.62 14.77,46.4 14.77,56.18 v16.37,57.78 | 26.33,58.85 26.33,57.96 25.97,57.6 GATES.12 | 26.33,58.85 26.51,59.02 28.28,59.02 | 28.28,59.02 28.28,57.6 GATES.14 | 28.28,59.02 28.28,63.65 GATES.1 | v25.62,59.38 26.15,58.85 26.33,58.85 | MAX3232.16 55.31,12.08 55.31,12.26 59.4,12.26 C3.1 59.58,12.44 59.58,19.02 v60.82,20.26 | 52.82,63.11 LOGIC.41 | 56.02,52.45 LOGIC.32 55.84,52.45 53.71,52.45 52.82,53.34 52.82,56.53 | 52.82,56.53 52.82,62.94 LOGIC.41 | 54.69,65.69 52.82,63.82 52.82,63.29 LOGIC.41 | 54.69,65.69 56.73,67.74 56.73,73.07 63.49,73.07 v65.09,71.47 65.09,71.29 66.33,70.05 66.33,20.98 69.35,20.98 C1.+ | 54.69,65.69 51.58,68.8 51.58,73.07 38.95,73.07 37.71,71.83 ADAPTER.20 | v37.71,56.18 v35.75,58.14 | v52.64,56.53 52.82,56.53 | v44.64,56.18 44.64,52.27 45,51.91 45,47.47 45.35,47.11 LOGIC.21
  Bottom 0.406: v17.08,33.07 17.26,32.89 41.62,32.89 41.97,32.53 TMS9902.18 42.15,32.53 v44.82,35.2 | v16.37,57.78 17.44,58.85 22.42,58.85 22.95,58.31 24.55,58.31 v25.62,59.38 25.79,59.38 27.04,58.14 v35.75,58.14 | v60.82,20.26 68.82,20.26 69.35,20.8 C1.+ | v65.09,71.47 67.93,71.47 73.98,65.43 POWER.2 | v37.71,56.18 38.06,56.53 44.64,56.53 | v52.64,56.53 44.64,56.53 | v44.64,56.18 44.64,56.53
XOUT  (via drill 0.61)
  Top 0.254: v52.64,5.51 52.64,5.69 55.13,5.69 MAX3232.11 | v43.75,8.88 43.57,9.06 43.57,19.91 44.46,20.8 44.46,24.71 TMS9902.2
  Bottom 0.254: v52.64,5.51 47.13,5.51 v43.75,8.88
